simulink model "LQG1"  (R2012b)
settings: Solver=ode45  StartTime=0.0  StopTime=50  RelTol=1e-3
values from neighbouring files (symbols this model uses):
  Kest1 = kalman(sys1,vnd,vny),    [LQG_1.m]
  sys1 = ss(H1)    [kalman_11.m]    (also in kalman_12.m; kalman_13.m = ss(H1*H2); kalman_2.m; kalman_3.m)
  vnd = 1e-4    (= 0.0001)    [kalman_1.m]    (also in kalman_10.m; kalman_11.m; kalman_12.m; kalman_13.m = 0.01)
  vny = 1e-6    (= 1e-06)    [kalman_1.m]    (also in kalman_10.m; kalman_11.m = ', num2str(vny),' )']); kalman_12.m = ', num2str(vny),' )']); kalman_13.m = ', num2str(vny),' )']))
undefined symbols (not defined in the file or in its folder): K1
libraries: simulink x2, dsparch4 x1

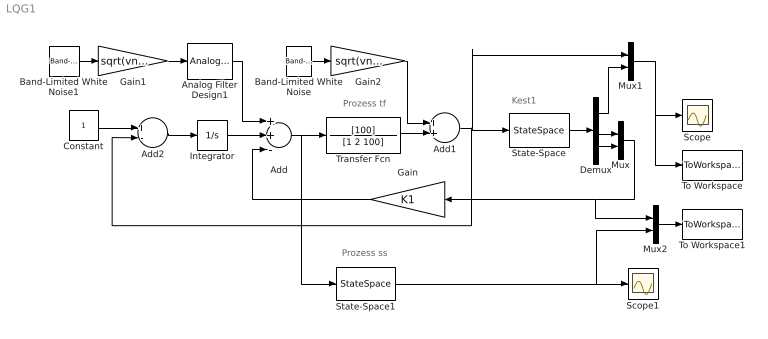
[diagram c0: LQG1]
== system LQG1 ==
  note: Prozess ss
  note: Prozess tf
  note: Kest1
  Add : Sum  Inputs=++-
  Add1 : Sum
  Add2 : Sum  Inputs=+-
  Analog Filter Design1 : dsparch4/Analog Filter Design  method=Butterworth  filttype=Lowpass  N=8  Wlo=30  Whi=80  Rp=2  Rs=40
  Band-Limited White Noise : simulink/Sources/Band-Limited White Noise  Cov=[0.01]  Ts=0.01  seed=[23341]
  Band-Limited White Noise1 : simulink/Sources/Band-Limited White Noise  Cov=[0.01]  Ts=0.01  seed=[296441]
  Constant : Constant
  Demux : Demux  Outputs=3
  Gain : Gain  Gain=K1  Multiplication=Matrix(K*u)
  Gain1 : Gain  Gain=sqrt(vnd)
  Gain2 : Gain  Gain=sqrt(vny)
  Integrator : Integrator
  Mux : Mux  Inputs=2
  Mux1 : Mux  Inputs=2
  Mux2 : Mux  Inputs=2
  Scope : Scope
  Scope1 : Scope
  State-Space : StateSpace  A=Kest1.a  B=Kest1.b  C=Kest1.c  D=Kest1.d
  State-Space1 : StateSpace  A=sys1.a  B=sys1.b  C=eye(2,2)  D=[0;0]
  To Workspace : ToWorkspace  VariableName=y  SaveFormat=Structure With Time
  To Workspace1 : ToWorkspace  VariableName=y1  SaveFormat=Structure With Time
  Transfer Fcn : TransferFcn  Numerator=[100]  Denominator=[1 2 100]
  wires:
  Band-Limited White Noise1/1 -> Gain1/1
  Gain1/1 -> Analog Filter Design1/1
  State-Space/1 -> Demux/1
  Demux/2 -> Mux/1
  Demux/3 -> Mux/2
  Mux/1 -> Mux2/1, Gain/1
  Transfer Fcn/1 -> Add1/2
  Band-Limited White Noise/1 -> Gain2/1
  Gain/1 -> Add/3
  Add2/1 -> Integrator/1
  Constant/1 -> Add2/1
  Gain2/1 -> Add1/1
  Add1/1 -> Mux1/1, Add2/2, State-Space/1
  Integrator/1 -> Add/2
  Demux/1 -> Mux1/2
  Mux1/1 -> To Workspace/1, Scope/1
  Mux2/1 -> To Workspace1/1
  State-Space1/1 -> Mux2/2, Scope1/1
  Add/1 -> State-Space1/1, Transfer Fcn/1
  Analog Filter Design1/1 -> Add/1
